(* Logix 5000 AddOnInstructionDefinition export Banner_Q20EAF_PD_v4; software revision 33.00 *)

TYPE Banner_Q20EAF_PDI_v4 :   // Process Data for a Q20 ABS sensors. This will include event information.
STRUCT
   Output_State : SINT;   // 0 = Inactive, 1 = Active
   Marginal_Signal : SINT;   // 0 = Normal, 1 = Marginal.
END_STRUCT
END_TYPE

ADD_ON_INSTRUCTION Banner_Q20EAF_PD_v4   (* revision 4.0, vendor Banner Engineering *)
// Take raw process data and convert it to usable values.
VAR_IN_OUT
   Process_Data : Banner_Q20EAF_PDI_v4; {required}
END_VAR
VAR_INPUT
   SINTO : SINT; {required}
   SINT1 : SINT; {required}
END_VAR
VAR
   Temp_Byte : SINT[4]; {access None}
END_VAR

ROUTINE Logic   (* ladder *)
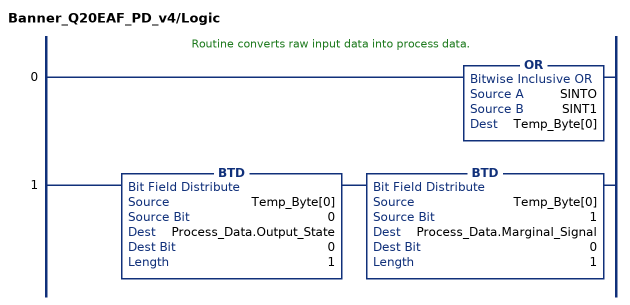
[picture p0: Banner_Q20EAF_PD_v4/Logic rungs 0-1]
   // Routine converts raw input data into process data.
   0: OR(SINTO,SINT1,Temp_Byte[0]);
   1: BTD(Temp_Byte[0],0,Process_Data.Output_State,0,1)BTD(Temp_Byte[0],1,Process_Data.Marginal_Signal,0,1);
END_ROUTINE
END_ADD_ON_INSTRUCTION
